PROGRAM MAIN
VAR
	bSwitchMultiCycle				:	BOOL;
	stEl5131						:	ST_EL5131;
	{attribute 'displaymode':='bin'}
	stEL5131Setting					:	ST_EL5131_Setting :=   (SetDigitalOutput		:= FALSE,
																(*EnableThresholdsOutput:= FALSE,*)
																SetTristate				:= FALSE,
																DisableThresholdsCw		:= FALSE,
																DisableThresholdsCcw	:= TRUE);
	//==========================================================================================
	// Multi
	fbEL5131_MultiCycle				:	FB_EL5131_MultiCycle;
	cNum							:	UDINT := 10;
	//==========================================================================================
	// Single 由于主程序没有调用，要先声明初始化中的变量
	fbEL5131_SingleCycle			:	FB_EL5131_SingleCycle:=(nDistWindow		:= 5,
																stEl5131		:= stEl5131,
																OutputOption	:= 2#0000_0001,
																InputOption		:= stEL5131Setting);
	nState							:	INT;
	bInit							:	BOOL;
	bReset							:	BOOL;
	bSetRefPos						:	BOOL;
	rSetRefPos						:	LREAL;
	bRun							:	BOOL;
	
END_VAR
VAR PERSISTENT
	// Multi-Cycle 
	arData							:	ARRAY[1..20] OF ST_EL5131_CamData;
	nActNum							:	UDINT :=5;
	// Single-Cycle
	arDataSingle					:	ARRAY[1..8] OF ST_EL5131_CamData;
END_VAR


IF bSwitchMultiCycle
THEN 
	// MultiCycle
	fbEL5131_MultiCycle(
		stEl5131:= stEl5131, // reference to ,link MAIN.stEl5131
		bReset:= , 
		bExecute:= , 
		bSetRefPos:= , 
		rRefPos:= , 
		rScaleFactor:= , 
		OutputOption:= , 
		InputOption:= stEL5131Setting, // default:DisableThresholdsCcw	:= TRUE
		pstEL5131_CamData:= ADR(arData),
		nSize:= SIZEOF(arData),
		cNum:= cNum,
		nActNum:= nActNum,// PERSISTENT
		bBusy=> , 
		bDone=> , 
		bError=> , 
		nErrId=> , 
		sErr=> );
ELSE
	// SingleCycle
	fbEL5131_SingleCycle.Cyclic();
	IF bReset 
	AND_THEN NOT fbEL5131_SingleCycle.Reset(TRUE)
	THEN 
		bReset						:= FALSE;
	END_IF
	
	IF bSetRefPos 
	AND_THEN NOT fbEL5131_SingleCycle.SetRefPos(TRUE,rSetRefPos)
	THEN 
		bSetRefPos					:= FALSE;
	END_IF
	
	IF bInit 
	AND_THEN NOT fbEL5131_SingleCycle.Init(TRUE)
	THEN 
		bInit						:= FALSE;	
	END_IF
	
	IF bRun 
	AND_THEN NOT fbEL5131_SingleCycle.Run(TRUE,ADR(arDataSingle),SIZEOF(arDataSingle)) // 1<=arDataSingle<=8
	THEN 
		bRun						:= FALSE;
	END_IF

END_IF

END_PROGRAM
